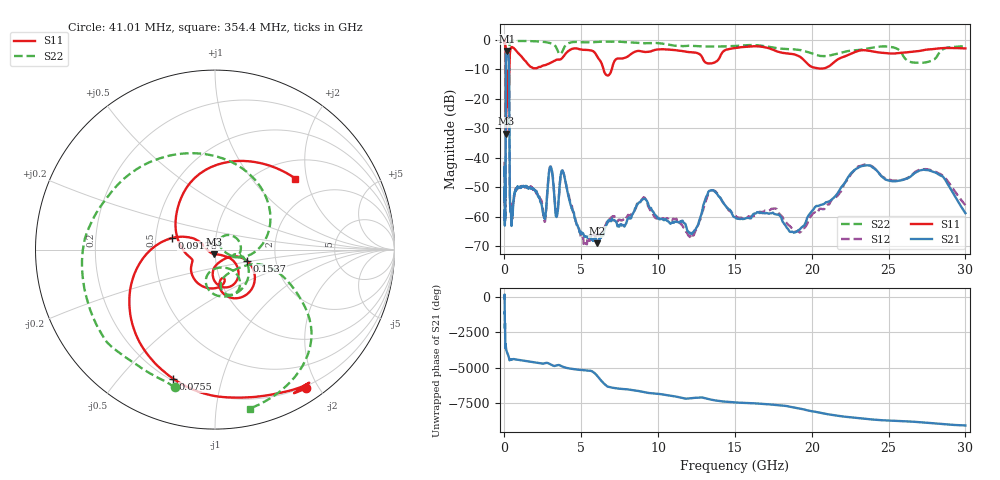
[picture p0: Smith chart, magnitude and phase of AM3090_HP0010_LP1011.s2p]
! Date/Time: Thu, Feb 28, 2019 1:55 PM
! Network Analyzer: Agilent Technologies E8364B Rev: A.07.50.67
! Sweep from 0.010 to 30.000 GHz, 1601 Points, Sweep Type: LOG
! Power Supply: 5.022 V, 0.002 A
# Hz S DB R 50
!freq MagS11 AngS11 MagS21 AngS21 MagS12 AngS12 MagS22 AngS22
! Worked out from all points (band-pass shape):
!   1601 points, 10 MHz to 30 GHz, reference 50 ohm
!   highest |S21| = -3.74 dB at 152.9 MHz (marker M1); lowest = -68.9 dB at 6.049 GHz (marker M2)
!   |S21| within 3 dB of the highest: 101.9 MHz to 284.2 MHz (182.3 MHz wide, 94.4 % of centre)
!   lowest |S11| = -31.8 dB at 99.92 MHz (marker M3), VSWR 1.05, Z = 49.3 - j2.46 ohm
!   |S11| at or under -10 dB: 90.65 MHz to 314.5 MHz (223.9 MHz wide, 111 % of centre); 6.451 GHz to 6.979 GHz (528.4 MHz wide, 7.87 % of centre)
!   |S22| runs from -29.5 to -0.2 dB; largest |S21 - S12| = 0.013
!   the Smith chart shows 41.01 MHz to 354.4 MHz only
!   S11 on the Smith chart (normalised r, x): 41.01 MHz: 0.17, -1.84; 75.5 MHz: 0.21, -0.71; 91.78 MHz: 0.61, +0.08; 153.7 MHz: 1.41, -0.18; 354.4 MHz: 1.39, +1.71
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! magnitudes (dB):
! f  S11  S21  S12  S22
! 10 MHz  -0.2  -46.1  -41.3  -0.6
! 38.04 MHz  -0.5  -61.2  -57.8  -1.7
! 41.01 MHz  -0.7  -59.0  -60.3  -1.9
! 75.5 MHz  -2.4  -46.0  -48.9  -4.4
! 91.78 MHz  -12.1  -14.8  -14.7  -12.1
! 99.92 MHz  -31.8  -7.4  -7.4  -28.8
! 115.5 MHz  -13.3  -4.9  -4.9  -18.3
! 144.7 MHz  -20.8  -3.8  -3.8  -19.2
! 152.9 MHz  -15.0  -3.7  -3.7  -16.6
! 153.7 MHz  -14.6  -3.7  -3.7  -16.4
! 288.7 MHz  -16.2  -7.4  -7.3  -15.4
! 354.4 MHz  -4.5  -53.4  -53.8  -0.9
! 550.5 MHz  -2.6  -56.7  -55.6  -0.3
! 2.084 GHz  -9.6  -51.4  -51.7  -0.5
! 3.017 GHz  -7.7  -43.0  -42.9  -1.1
! 3.402 GHz  -6.7  -59.9  -59.2  -2.9
! 3.798 GHz  -5.9  -44.5  -44.6  -3.5
! 6.049 GHz  -5.8  -68.9  -66.3  -0.6
! 7.926 GHz  -5.9  -62.1  -60.2  -0.8
! 19.03 GHz  -5.2  -65.0  -64.9  -3.3
! 23.36 GHz  -3.5  -42.7  -42.4  -3.1
! 30 GHz  -2.9  -58.7  -56.0  -2.2
